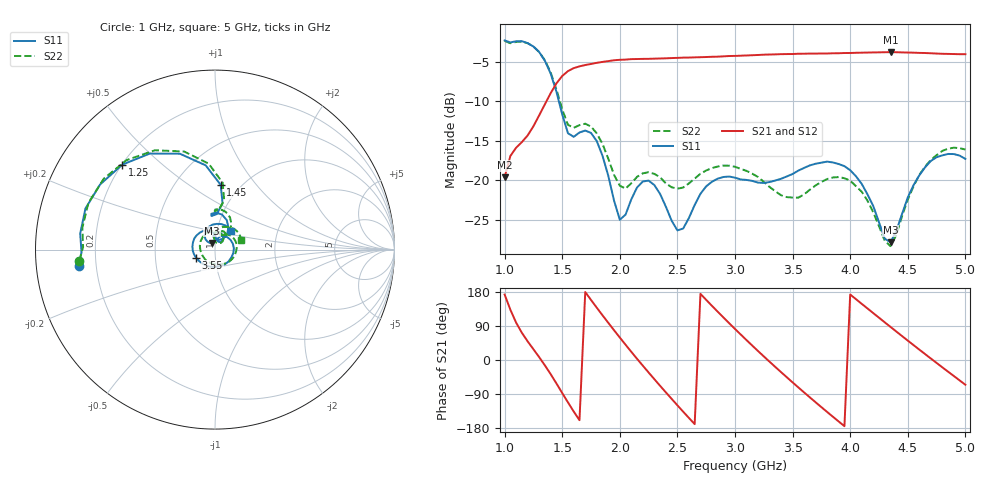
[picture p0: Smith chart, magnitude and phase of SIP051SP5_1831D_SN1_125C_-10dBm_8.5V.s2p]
# GHz  S  dB  R  50
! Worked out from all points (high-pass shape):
!   81 points, 1 GHz to 5 GHz, reference 50 ohm
!   highest |S21| = -3.81 dB at 4.35 GHz (marker M1); lowest = -19.6 dB at 1 GHz (marker M2)
!   |S21| within 3 dB of the highest: 1.501 GHz to end of sweep
!   lowest |S11| = -27.9 dB at 4.35 GHz (marker M3), VSWR 1.08, Z = 48.2 + j3.56 ohm
!   |S11| at or under -10 dB: 1.471 GHz to end of sweep
!   |S22| runs from -28.3 to -2.4 dB; largest |S21 - S12| = 0.0021
!   S11 on the Smith chart (normalised r, x): 1 GHz: 0.13, -0.06; 1.25 GHz: 0.20, +0.38; 1.45 GHz: 0.81, +0.68; 3.55 GHz: 0.81, -0.08; 5 GHz: 1.17, +0.24
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1  -2.33 -173.1  -19.62 172.8  -19.60 172.5  -2.39 -175.2
1.25  -3.09 137.5  -13.18 28.4  -13.17 28.3  -3.09 134.6
1.45  -8.82 85.0  -7.75 -61.9  -7.75 -61.9  -8.52 83.5
1.55  -14.06 87.2  -6.20 -111.9  -6.20 -112.0  -13.00 84.4
1.7  -13.72 88.6  -5.43 179.4  -5.43 179.4  -12.85 82.8
1.85  -16.92 58.3  -5.04 117.9  -5.03 117.9  -15.41 57.3
1.95  -22.58 53.6  -4.83 78.6  -4.84 78.6  -19.33 53.0
2  -25.00 71.3  -4.77 59.3  -4.75 59.3  -20.70 60.6
2.15  -20.91 92.4  -4.67 3.1  -4.67 3.1  -19.57 73.5
2.35  -21.74 56.7  -4.61 -68.2  -4.59 -68.1  -19.64 55.1
2.5  -26.35 59.9  -4.53 -119.6  -4.52 -119.6  -21.07 53.8
2.7  -21.73 66.8  -4.44 174.6  -4.42 174.6  -19.19 49.4
2.85  -19.80 31.6  -4.38 127.4  -4.36 127.4  -18.27 29.5
3  -19.68 -10.6  -4.28 81.9  -4.27 81.9  -18.30 4.0
3.25  -20.35 -84.1  -4.12 9.5  -4.13 9.5  -20.21 -50.8
3.55  -18.79 -156.4  -4.00 -72.4  -4.01 -72.4  -22.20 -156.1
3.7  -17.92 171.8  -3.99 -111.6  -3.98 -111.6  -20.66 150.2
4  -18.74 112.9  -3.91 172.9  -3.92 172.9  -20.06 75.7
4.2  -23.26 86.3  -3.84 123.8  -3.85 123.8  -24.06 47.3
4.35  -27.85 114.6  -3.81 87.3  -3.82 87.2  -28.35 74.2
4.7  -17.57 104.3  -3.94 3.9  -3.94 4.0  -17.43 70.3
5  -17.30 48.2  -4.06 -65.3  -4.07 -65.4  -16.12 20.5
